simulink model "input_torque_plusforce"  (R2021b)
settings: Solver=FixedStepAuto  StartTime=0.0  StopTime=2  FixedStep=1e-4  RelTol=1e-3
undefined symbols (not defined in the file or in its folder): BLDC, dynamics
libraries: fl_lib x21, nesl_utility x7, sdl_lib x1

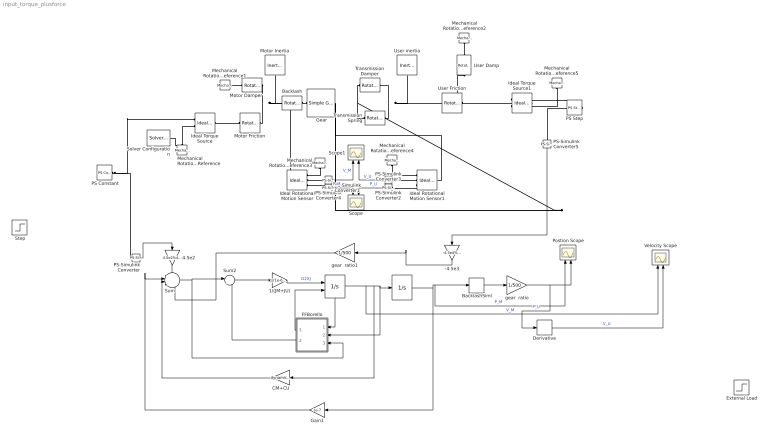
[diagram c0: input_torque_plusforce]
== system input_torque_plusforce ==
  " " : Integrator  ExternalReset=rising  ShowStatePort=on
  "  " : Integrator  UpperSaturationLimit=dynamics.ThUmax/dynamics.tau  LowerSaturationLimit=dynamics.ThUmin/dynamics.tau
  " Gear" : sdl_lib/Gears/Simple Gear  ratio=500  rotation_direction=sdl.enum.shaftOutputDirection.same  friction_model=sdl.enum.gear_efficiencies_load.off  T_noload=0.1 N*m  T_nom=5 N*m  efficiency_nom=0.8  efficiency=0.8  temperature_TLU=[280, 300, 320] K  load_TLU=[1, 5, 10] N*m  efficiency_TLU=[.95, .9, .85]  efficiency_TLU2=[.85, .8, .75; .95, .9, .85; .85, .8, .7]  w_thr=0.01 rad/s  pwr_thr=0.001 W  backlash_model=sdl.enum.backlashModel.Off  backlash_distance=1e-3 mm  x0=0 mm  r_base=0.1 m  hardstop_model=simscape.enum.hardstop.smooth  transition=1e-4 mm  backlash_stiffness=1e7 N/m  backlash_damping=1e6 N/(m/s)  e=0  v_tol=0.001 m/s  mu_visc=[0, 0] N*m/(rad/s)  enable_faults=simscape.enum.onoff.off  efficiency_fault=0.05  external_fault=simscape.enum.onoff.off  temporal_fault=simscape.enum.onoff.off  fault_time=5 s  fault_angles=pi / 12 rad  report_fault=simscape.enum.assert.action.none  thermal_mass=50 J/K  temperature_specify=off  temperature_priority=High  temperature=300 K  temperature_nominal_specify=off  temperature_nominal_unit=K  temperature_nominal_value=1
  -4.5e3 : Gain  Gain=-4.5e4%4.5e2
  1/(JM+JU) : Gain  Gain=1/(1e-6)%1/(dynamics.JM+dynamics.JU)
  4.5e2 : Gain  Gain=4.5e2%4.5e2
  Backlash : fl_lib/Mechanical/Rotational Elements/Rotational Hard Stop  upper_bnd=1%1e-10%1 deg  lower_bnd=-1%1e-11%-1 deg  stiff_up=1e6 N*m/rad  stiff_low=1e6 N*m/rad  D_up=0.01 N*m/(rad/s)  D_low=0.01 N*m/(rad/s)  model=simscape.enum.hardstop.smooth  transition=0.001 rad  w_specify=off  w_priority=None  w=0 rad/s  w_nominal_specify=off  w_nominal_unit=rad/s  w_nominal_value=1  t_specify=off  t_priority=None  t=0 N*m  t_nominal_specify=off  t_nominal_unit=N*m  t_nominal_value=1  phi_specify=off  phi_priority=High  phi=0 rad  phi_nominal_specify=off  phi_nominal_unit=rad  phi_nominal_value=1
  BacklashSiml : Backlash  BacklashWidth=1/57
  CM+CU : Gain  Gain=dynamics.CM+dynamics.CU
  Derivative : Derivative
  External Load : Step  Time=1.4  After=-8.6e-5%-8.6e-5  SampleTime=0
  FFBorello : Subsystem
  Gain1 : Gain  Gain=1e-7
  Ideal Rotational Motion Sensor : fl_lib/Mechanical/Mechanical Sensors/Ideal Rotational Motion Sensor  wrap_angle=simscape.enum.onoff.off  offset=0 rad
  Ideal Rotational Motion Sensor1 : fl_lib/Mechanical/Mechanical Sensors/Ideal Rotational Motion Sensor  wrap_angle=simscape.enum.onoff.off  offset=0 rad
  Ideal Torque Source : fl_lib/Mechanical/Mechanical Sources/Ideal Torque Source
  Ideal Torque Source1 : fl_lib/Mechanical/Mechanical Sources/Ideal Torque Source
  Mechanical Rotational Reference{,1..5} (6 alike) : fl_lib/Mechanical/Rotational Elements/Mechanical Rotational Reference
  Motor Damper : fl_lib/Mechanical/Rotational Elements/Rotational Damper  D=1e-6 N*m/(rad/s)  w_specify=off  w_priority=None  w=0 rad/s  w_nominal_specify=off  w_nominal_unit=rad/s  w_nominal_value=1  t_specify=off  t_priority=None  t=0 N*m  t_nominal_specify=off  t_nominal_unit=N*m  t_nominal_value=1
  Motor Friction : fl_lib/Mechanical/Rotational Elements/Rotational Friction  brkwy_trq=dynamics.friction.FSTm*BLDC.TMM N*m  brkwy_vel=0.00001201 rad/s  Col_trq=dynamics.friction.FDTm*BLDC.TMM N*m  visc_coef=0 N*m/(rad/s)  w_specify=off  w_priority=None  w=0 rad/s  w_nominal_specify=off  w_nominal_unit=rad/s  w_nominal_value=1  t_specify=off  t_priority=None  t=0 N*m  t_nominal_specify=off  t_nominal_unit=N*m  t_nominal_value=1
  Motor Inertia : fl_lib/Mechanical/Rotational Elements/Inertia  inertia=dynamics.JM kg*m^2  num_ports=foundation.enum.numPorts2.one  w_specify=off  w_priority=High  w=0 rad/s  w_nominal_specify=off  w_nominal_unit=rad/s  w_nominal_value=1  t_specify=off  t_priority=None  t=0 N*m  t_nominal_specify=off  t_nominal_unit=N*m  t_nominal_value=1
  PS Constant : fl_lib/Physical Signals/Sources/PS Constant  constant=4e-4%0.0004 N*m
  PS Step : fl_lib/Physical Signals/Sources/PS Step  step_time=1.4 s  initial_value=0  final_value=-9.5e-5 N*m
  PS-Simulink Converter{,1..5} (6 alike) : nesl_utility/PS-Simulink Converter  PhysicalDomain=network_engine_domain  SubClassName=ps_output  LeftPortType=input  RightPortType=output  PseudoPeriodic=off  Frequencies=[]  Unit=inherit  AffineConversion=off
  Postion Scope : Scope  NumInputPorts=2
  Scope : Scope  NumInputPorts=2
  Scope1 : Scope  NumInputPorts=2
  Solver Configuration : nesl_utility/Solver Configuration  PhysicalDomain=network_engine_domain  SubClassName=solver  LeftPortType=input  RightPortType=generic  Tones=[]  Harmonics=[]  SimulateNoise=off  Profile=off  UseLocalSampling=off  EnableSwitchedLinearOptims=on  FrequencyDomain=off  UseCCode=off  RelTol=0.001  AbsTol=1e-06  MinStep=1e-09  ToWorkspace=off  RevertToSquareIcSolve=off  NumHomotopyIterations=100  PhasorMode=off  PhasorModeNumHarmonics=1  DoDC=off  ResidualTolerance=1e-09  UseLocalSolver=off  LocalSolverChoice=NE_BACKWARD_EULER_ADVANCER  LocalSolverSampleTime=0.001  DoFixedCost=off  MaxNonlinIter=3  MaxModeIter=2  ComputeImpulses=off  ImpulseIterations=2  LinearAlgebra=auto  EquationFormulation=NE_TIME_EF  DelaysMemoryBudget=1024  AutomaticFiltering=on  FilteringTimeConstant=0.001  PartitionStorageMethod=AS_NEEDED  PartitionMemoryBudget=1024  PartitionMethod=ROBUST
  Step : Step  Time=10  Before=0.17  After=-0.17  SampleTime=0
  Sum : Sum  Inputs=+---
  Sum2 : Sum  Inputs=|+-
  Transmission Damper : fl_lib/Mechanical/Rotational Elements/Rotational Damper  D=5e4%50000 N*m/(rad/s)  w_specify=off  w_priority=None  w=0 rad/s  w_nominal_specify=off  w_nominal_unit=rad/s  w_nominal_value=1  t_specify=off  t_priority=None  t=0 N*m  t_nominal_specify=off  t_nominal_unit=N*m  t_nominal_value=1
  Transmission Spring : fl_lib/Mechanical/Rotational Elements/Rotational Spring  spr_rate=1%0.00001%0.001 N*m/rad  w_specify=off  w_priority=None  w=0 rad/s  w_nominal_specify=off  w_nominal_unit=rad/s  w_nominal_value=1  t_specify=off  t_priority=None  t=0 N*m  t_nominal_specify=off  t_nominal_unit=N*m  t_nominal_value=1  phi_specify=off  phi_priority=High  phi=0 rad  phi_nominal_specify=off  phi_nominal_unit=rad  phi_nominal_value=1
  User Damp : fl_lib/Mechanical/Rotational Elements/Rotational Damper  D=1e-7 N*m/(rad/s)  w_specify=off  w_priority=None  w=0 rad/s  w_nominal_specify=off  w_nominal_unit=rad/s  w_nominal_value=1  t_specify=off  t_priority=None  t=0 N*m  t_nominal_specify=off  t_nominal_unit=N*m  t_nominal_value=1
  User Friction : fl_lib/Mechanical/Rotational Elements/Rotational Friction  brkwy_trq=dynamics.friction.FSTu*BLDC.TMM N*m  brkwy_vel=0.00001201 rad/s  Col_trq=dynamics.friction.FDTu*BLDC.TMM N*m  visc_coef=0 N*m/(rad/s)  w_specify=off  w_priority=None  w=0 rad/s  w_nominal_specify=off  w_nominal_unit=rad/s  w_nominal_value=1  t_specify=off  t_priority=None  t=0 N*m  t_nominal_specify=off  t_nominal_unit=N*m  t_nominal_value=1
  User inertia : fl_lib/Mechanical/Rotational Elements/Inertia  inertia=dynamics.JU kg*m^2  num_ports=foundation.enum.numPorts2.one  w_specify=off  w_priority=High  w=0 rad/s  w_nominal_specify=off  w_nominal_unit=rad/s  w_nominal_value=1  t_specify=off  t_priority=None  t=0 N*m  t_nominal_specify=off  t_nominal_unit=N*m  t_nominal_value=1
  Velocity Scope : Scope  NumInputPorts=2
  gear  ratio : Gain  Gain=1/500
  gear  ratio1 : Gain  Gain=1/500
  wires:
  PS-Simulink Converter1/1 -> Scope/1  "P_M"
  PS-Simulink Converter3/1 -> Scope/2  "P_U"
  PS-Simulink Converter4/1 -> Scope1/1  "V_M"
  PS-Simulink Converter2/1 -> Scope1/2  "V_U"
  1/(JM+JU)/1 -> " "/1  "D2XJ"
  Sum/1 -> FFBorello/3(Act Torque), Sum2/1
  Gain1/1 -> Sum/2
  Sum2/1 -> 1/(JM+JU)/1
  FFBorello/1(Reset_DXJ) -> " "/2
  " "/1 -> Velocity Scope/1, CM+CU/1, "  "/1, FFBorello/2(DXJ)  "V_M"
  FFBorello/2(TF) -> Sum2/2
  " "/State -> FFBorello/1(DXJ SP)
  "  "/1 -> Gain1/1, Postion Scope/1, BacklashSiml/1  "P_M"
  gear  ratio/1 -> Postion Scope/2, Derivative/1  "P_U"
  PS-Simulink Converter/1 -> 4.5e2/1
  4.5e2/1 -> Sum/1
  BacklashSiml/1 -> gear  ratio/1
  Derivative/1 -> Velocity Scope/2  "V_U"
  gear  ratio1/1 -> Sum/4
  -4.5e3/1 -> gear  ratio1/1
  CM+CU/1 -> Sum/3
  PS-Simulink Converter5/1 -> -4.5e3/1
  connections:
  PS Constant/RConn1 -- Ideal Torque Source/RConn1 -- PS-Simulink Converter/LConn1
  Mechanical Rotational Reference/LConn1 -- Solver Configuration/RConn1 -- Ideal Torque Source/RConn2
  Motor Friction/LConn1 -- Ideal Torque Source/LConn1
  Motor Friction/RConn1 -- Ideal Rotational Motion Sensor/LConn1 -- Backlash/LConn1 -- Motor Inertia/LConn1 -- Motor Damper/RConn1
  Mechanical Rotational Reference1/LConn1 -- Motor Damper/LConn1
  Transmission Damper/LConn1 -- Ideal Rotational Motion Sensor1/LConn1 -- " Gear"/RConn1 -- Transmission Spring/LConn1
  Transmission Damper/RConn1 -- User Friction/LConn1 -- User inertia/LConn1 -- Transmission Spring/RConn1
  User Friction/RConn1 -- User Damp/RConn1 -- Ideal Torque Source1/LConn1
  Mechanical Rotational Reference2/LConn1 -- User Damp/LConn1
  Backlash/RConn1 -- " Gear"/LConn1
  PS-Simulink Converter1/LConn1 -- Ideal Rotational Motion Sensor/RConn3
  Ideal Rotational Motion Sensor1/RConn3 -- PS-Simulink Converter3/LConn1
  Mechanical Rotational Reference3/LConn1 -- Ideal Rotational Motion Sensor/RConn1
  Mechanical Rotational Reference4/LConn1 -- Ideal Rotational Motion Sensor1/RConn1
  PS-Simulink Converter4/LConn1 -- Ideal Rotational Motion Sensor/RConn2
  PS-Simulink Converter2/LConn1 -- Ideal Rotational Motion Sensor1/RConn2
  Mechanical Rotational Reference5/LConn1 -- Ideal Torque Source1/RConn2
  PS Step/RConn1 -- PS-Simulink Converter5/LConn1 -- Ideal Torque Source1/RConn1

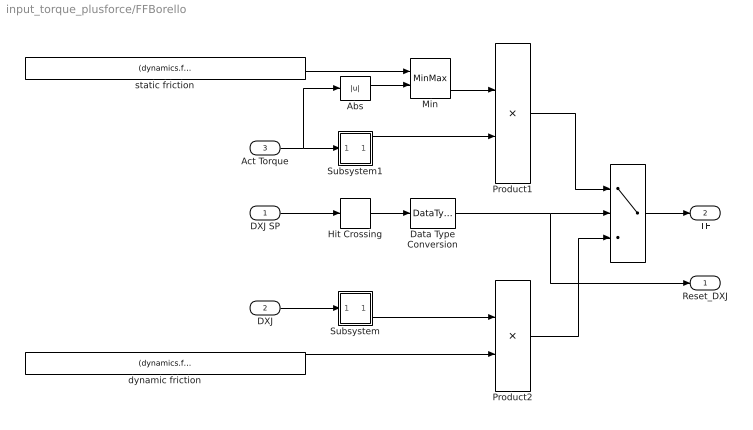
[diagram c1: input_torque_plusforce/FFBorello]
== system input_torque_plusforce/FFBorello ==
  DXJ SP : Inport
  DXJ : Inport  Port=2
  Act Torque : Inport  Port=3
  "   " : Switch  Threshold=0.5
  Abs : Abs
  Data Type Conversion : DataTypeConversion  OutDataTypeStr=double
  Hit Crossing : HitCross
  Min : MinMax  Inputs=2  InputSameDT=on  SaturateOnIntegerOverflow=on
  Product1 : Product  InputSameDT=on  RndMeth=Zero  SaturateOnIntegerOverflow=on
  Product2 : Product  InputSameDT=on  RndMeth=Zero  SaturateOnIntegerOverflow=on
  Subsystem : Subsystem
  Subsystem1 : Subsystem
  dynamic friction : Constant  Value=(dynamics.friction.FDTm+dynamics.friction.FDTu)*BLDC.TMM
  static friction : Constant  Value=(dynamics.friction.FSTm+dynamics.friction.FSTu)*BLDC.TMM
  Reset_DXJ : Outport
  TF : Outport  Port=2
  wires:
  Product2/1 -> "   "/3
  DXJ/1 -> Subsystem/1(In1)
  "   "/1 -> TF/1
  Product1/1 -> "   "/1
  Min/1 -> Product1/1
  Act Torque/1 -> Subsystem1/1(In1), Abs/1
  Abs/1 -> Min/2
  Hit Crossing/1 -> Data Type Conversion/1
  Subsystem/1(Out1) -> Product2/1
  Subsystem1/1(Out1) -> Product1/2
  Data Type Conversion/1 -> "   "/2, Reset_DXJ/1
  DXJ SP/1 -> Hit Crossing/1
  static friction/1 -> Min/1
  dynamic friction/1 -> Product2/2

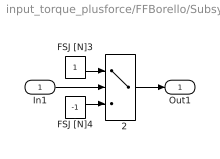
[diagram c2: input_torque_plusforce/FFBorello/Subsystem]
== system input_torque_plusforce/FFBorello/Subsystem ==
  In1 : Inport
  "   2" : Switch
  FSJ [N]3 : Constant
  FSJ [N]4 : Constant  Value=-1
  Out1 : Outport
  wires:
  FSJ [N]3/1 -> "   2"/1
  FSJ [N]4/1 -> "   2"/3
  In1/1 -> "   2"/2
  "   2"/1 -> Out1/1

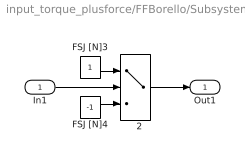
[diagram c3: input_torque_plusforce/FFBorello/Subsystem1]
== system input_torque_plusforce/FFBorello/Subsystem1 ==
  In1 : Inport
  "   2" : Switch
  FSJ [N]3 : Constant
  FSJ [N]4 : Constant  Value=-1
  Out1 : Outport
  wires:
  FSJ [N]3/1 -> "   2"/1
  FSJ [N]4/1 -> "   2"/3
  In1/1 -> "   2"/2
  "   2"/1 -> Out1/1
